FUNCTION_BLOCK AnalogConverter
VAR_INPUT
	AnalogRdValue_In_Int: INT;
	AnalogResMin_In_Int: INT;
	AnalogResMax_In_Int: INT;
	AnalogPhyMin_In_Real: REAL;
	AnalogPhyMax_In_Real: REAL;
	AnalogRdOffset_In_Real: REAL;
END_VAR
VAR_OUTPUT
	ActRdValue_Out_Real: REAL;
END_VAR
VAR
END_VAR

//模拟量输入限定范围
AnalogRdValue_In_Int := LIMIT(	AnalogResMin_In_Int , AnalogRdValue_In_Int , AnalogResMax_In_Int );

ActRdValue_Out_Real := 
	(	INT_TO_REAL (AnalogRdValue_In_Int)  - INT_TO_REAL (AnalogResMin_In_Int) ) / (	INT_TO_REAL (AnalogResMax_In_Int ) - INT_TO_REAL (AnalogResMin_In_Int) ) * 
	(	AnalogPhyMax_In_Real - AnalogPhyMin_In_Real ) + AnalogPhyMin_In_Real + AnalogRdOffset_In_Real ;

END_FUNCTION_BLOCK
